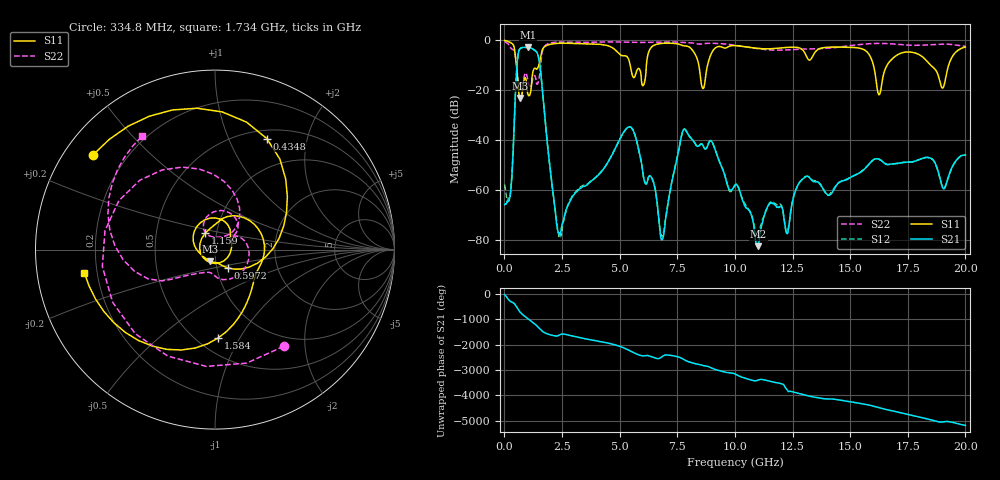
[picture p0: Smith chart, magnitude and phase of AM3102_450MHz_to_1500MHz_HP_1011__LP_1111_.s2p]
!Agilent Technologies,E8364B,MY43040894,A.07.50.67
!Agilent E8364B: A.07.50.67
!Date: Thursday, January 11, 2018 06:26:55
!Correction: S11(Full 2 Port(1,2))
!S21(Full 2 Port(1,2))
!S12(Full 2 Port(1,2))
!S22(Full 2 Port(1,2))
!S2P File: Measurements: S11, S21, S12, S22:
# Hz S  dB  R 50
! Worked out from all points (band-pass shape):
!   1601 points, 10 MHz to 20 GHz, reference 50 ohm
!   highest |S21| = -2.80 dB at 1.022 GHz (marker M1); lowest = -82.6 dB at 11.02 GHz (marker M2)
!   |S21| within 3 dB of the highest: 595.2 MHz to 1.453 GHz (857.9 MHz wide, 83.8 % of centre)
!   lowest |S11| = -23.2 dB at 697.2 MHz (marker M3), VSWR 1.15, Z = 47 - j6.07 ohm
!   |S11| at or under -10 dB: 524.5 MHz to 1.49 GHz (965.8 MHz wide, 95.9 % of centre); 5.459 GHz to 6.16 GHz (701.5 MHz wide, 12.1 % of centre); 18.5 GHz to 19.27 GHz (777 MHz wide, 4.11 % of centre)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
!   |S22| runs from -23.2 to -0.5 dB; largest |S21 - S12| = 0.0012
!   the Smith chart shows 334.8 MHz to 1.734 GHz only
!   S11 on the Smith chart (normalised r, x): 334.8 MHz: 0.08, +0.34; 434.8 MHz: 0.60, +1.39; 597.2 MHz: 1.13, -0.24; 1.159 GHz: 0.88, +0.16; 1.584 GHz: 0.63, -0.82; 1.734 GHz: 0.15, -0.09
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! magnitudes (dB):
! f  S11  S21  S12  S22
! 10 MHz  -0.1  -65.9  -57.9  -0.5
! 334.8 MHz  -1.3  -53.1  -52.4  -3.6
! 434.8 MHz  -3.3  -31.7  -31.5  -4.4
! 597.2 MHz  -18.0  -5.7  -5.7  -17.3
! 697.2 MHz  -23.2  -3.2  -3.2  -23.2
! 1.022 GHz  -21.7  -2.8  -2.8  -16.2
! 1.159 GHz  -19.5  -3.1  -3.1  -18.0
! 1.584 GHz  -6.1  -13.6  -13.6  -9.3
! 1.734 GHz  -2.6  -28.9  -28.9  -2.5
! 2.371 GHz  -1.2  -77.1  -79.1  -0.7
! 3.346 GHz  -1.4  -59.1  -58.6  -0.8
! 5.457 GHz  -9.9  -34.7  -34.8  -0.8
! 6.682 GHz  -1.4  -70.1  -69.9  -0.7
! 6.882 GHz  -1.2  -79.4  -78.0  -0.7
! 7.806 GHz  -2.2  -35.6  -35.6  -0.9
! 8.618 GHz  -19.4  -42.3  -42.3  -1.4
! 10.01 GHz  -2.1  -58.2  -58.0  -2.0
! 11.02 GHz  -3.3  -82.6  -78.3  -3.4
! 13.34 GHz  -6.9  -56.2  -56.0  -3.4
! 16.68 GHz  -9.0  -49.8  -49.8  -1.3
! 19.01 GHz  -19.2  -59.1  -59.0  -1.5
! 20 GHz  -2.7  -46.1  -46.1  -2.4
